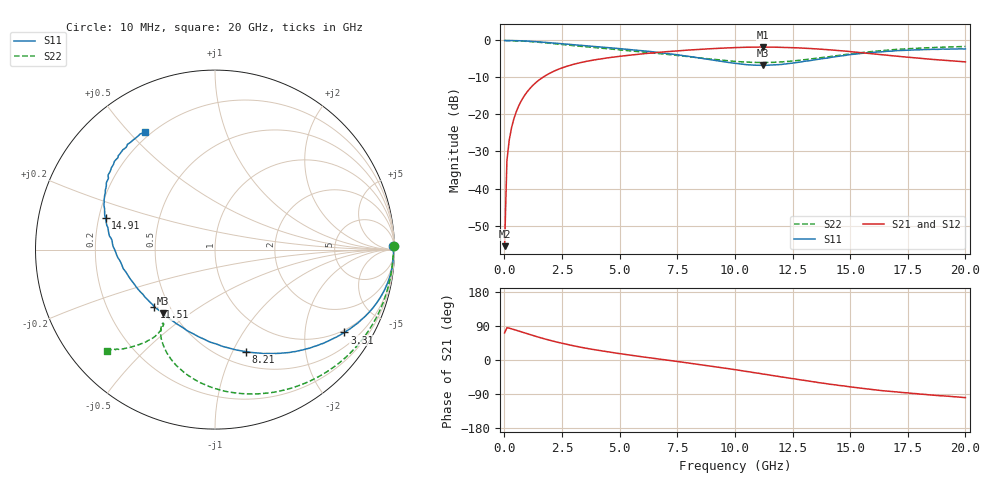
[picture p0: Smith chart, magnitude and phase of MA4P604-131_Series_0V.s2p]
! AWR Design Environment (9226) Thu Aug 19 15:08:55 2021
! Document = '0V'
! nPorts: 2, nXvals: 201
# GHz S DB R 50
!Freq DBS11 AngS11 DBS21 AngS21 DBS12 AngS12 DBS22 AngS22
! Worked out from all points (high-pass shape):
!   201 points, 10 MHz to 20 GHz, reference 50 ohm
!   highest |S21| = -1.81 dB at 11.21 GHz (marker M1); lowest = -55.6 dB at 10 MHz (marker M2)
!   |S21| within 3 dB of the highest: 4.379 GHz to 17.95 GHz (13.58 GHz wide, 122 % of centre)
!   lowest |S11| = -6.8 dB at 11.21 GHz (marker M3), VSWR 2.69, Z = 22 - j19.7 ohm
!   |S11| at or under -10 dB: nowhere
!   |S22| runs from -6.0 to 0.0 dB; largest |S21 - S12| = 0.024
!   S11 on the Smith chart (normalised r, x): 10 MHz: 25, +80; 3.31 GHz: 0.92, -3.17; 8.21 GHz: 0.64, -1.13; 11.51 GHz: 0.41, -0.34; 14.91 GHz: 0.23, +0.13; 20 GHz: 0.18, +0.56
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0.01  -0.06 1.3  -55.56 71.5  -52.06 65.0  -0.03 1.0
0.11  -0.04 -1.4  -32.52 85.0  -32.51 85.1  -0.07 -3.1
0.21  -0.05 -2.6  -26.95 84.1  -26.95 84.1  -0.08 -6.0
0.31  -0.05 -3.8  -23.61 82.3  -23.61 82.4  -0.09 -8.8
0.41  -0.07 -5.0  -21.22 80.5  -21.22 80.5  -0.11 -11.6
0.61  -0.10 -7.4  -17.86 76.6  -17.87 76.7  -0.15 -17.1
1.01  -0.21 -11.9  -13.73 69.0  -13.74 69.2  -0.28 -27.9
1.61  -0.46 -18.3  -10.22 58.0  -10.22 58.3  -0.58 -42.9
2.41  -0.87 -25.6  -7.65 45.4  -7.65 45.9  -1.06 -60.0
3.31  -1.35 -32.6  -6.00 33.7  -5.99 34.4  -1.61 -75.4
3.41  -1.40 -33.3  -5.87 32.6  -5.85 33.3  -1.66 -76.9
4.91  -2.18 -43.7  -4.37 17.6  -4.35 18.4  -2.50 -95.4
6.71  -3.28 -57.4  -3.23 2.6  -3.17 3.5  -3.55 -110.9
8.21  -4.53 -73.2  -2.53 -9.8  -2.48 -8.8  -4.56 -119.9
10.01  -6.21 -102.4  -1.96 -25.6  -1.90 -24.3  -5.69 -125.1
11.21  -6.77 -129.5  -1.81 -36.9  -1.76 -35.5  -5.99 -125.1
11.51  -6.66 -136.6  -1.83 -39.8  -1.76 -38.4  -5.96 -124.6
13.41  -5.30 -175.2  -2.25 -57.4  -2.16 -56.1  -4.94 -124.1
14.91  -3.95 163.9  -2.98 -70.1  -2.89 -68.9  -3.74 -127.3
16.71  -2.94 147.1  -4.09 -82.7  -4.03 -81.5  -2.60 -132.2
18.21  -2.48 136.0  -4.95 -90.5  -4.97 -90.0  -2.04 -135.4
20  -2.33 120.7  -5.81 -99.2  -5.99 -98.1  -1.65 -136.7
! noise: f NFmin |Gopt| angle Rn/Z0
0.01  0  1  0  2e-20
2.21  0  1  0  2e-20
4.41  0  1  0  2e-20
6.61  0  1  0  2e-20
8.81  0  1  0  2e-20
11.11  0  1  0  2e-20
13.31  0  1  0  2e-20
15.51  0  1  0  2e-20
17.71  0  1  0  2e-20
20  0  1  0  2e-20
